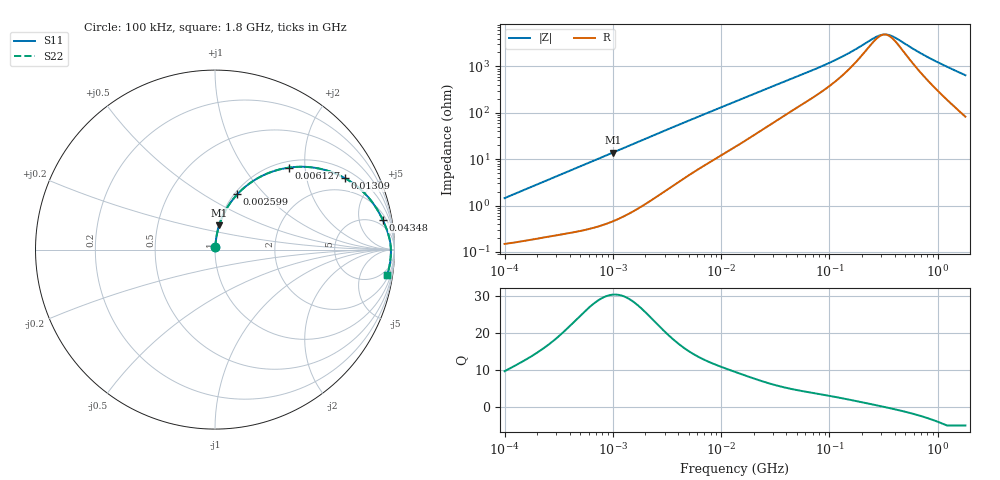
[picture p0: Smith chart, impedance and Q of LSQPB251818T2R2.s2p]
! LSQPB251818T2R2  S-PARAMETER MODEL  ( General Type )
! Model Generated by TAIYO YUDEN Corporation (http://www.ty-top.com)
! Version 2.0
! TAIYO YUDEN Control No. 100810NG19SB-FKC
! Copyright(c) 2009 TAIYO YUDEN CO.,LTD. All Rights Reserved.
! Product Description (link to TY-COMPAS)
! https://ds.yuden.co.jp/TYCOMPAS/or/detail?pn=LSQPB251818T2R2M&u=M
! Products Name : Inductors
! Characteristics :
!  Inductance : 2.2 uH , SRF(min) : 200 MHz , DC Resistance(max) : 0.156 Ohm
!  Rated Current : Saturation :1800 mA , Temp Rise : 1000 mA (40 degC)
!  Case Size : 2.5 x 1.8 / 0.098 x 0.071 [mm/inch] , Thickness : 1.8 / 0.071 [mm/inch]
!  (Conditions: Temperature = 25 degC , DC Bias Current/Voltage = 0A / 0V)
! External Node Assignments :
!  1  o---GGG---o  2
! GND o---------o GND
! Frequency Range : 0.1MHz  -  1800MHz  [ 402 STEP ]
# MHz S RI R 50
! Freq[MHz].  S11 Real  S11 Imag  S21 Real  S21 Imag  S12 Real  S12 Imag  S22 Real  S22 Imag
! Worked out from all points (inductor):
!   401 points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, 100 kHz to 1.8 GHz, reference 50 ohm
!   read as one part in series: L = 2.28 uH near 105 kHz
!   highest Q = 30.4 at 1 MHz (marker M1), where L = 2.21 uH
!   self-resonance near 322 MHz
!   S11 on the Smith chart (normalised r, x): 100 kHz: 1.00, +0.03; 2.599 MHz: 1.03, +0.71; 6.127 MHz: 1.12, +1.64; 13.09 MHz: 1.35, +3.38; 43.48 MHz: 3, +10; 1.8 GHz: 3, -13
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0.1  0.00169 0.0143  0.9983 -0.0143  0.9983 -0.0143  0.00169 0.0143
0.516129  0.00797 0.0712  0.992 -0.0712  0.992 -0.0712  0.00797 0.0712
0.999975  0.0232 0.1349  0.9768 -0.1349  0.9768 -0.1349  0.0232 0.1349
1.714072  0.0604 0.2207  0.9396 -0.2207  0.9396 -0.2207  0.0604 0.2207
2.59943  0.1241 0.308  0.8759 -0.308  0.8759 -0.308  0.1241 0.308
2.66389  0.1292 0.3134  0.8708 -0.3134  0.8708 -0.3134  0.1292 0.3134
3.942096  0.2367 0.3972  0.7633 -0.3972  0.7633 -0.3972  0.2367 0.3972
6.126528  0.41 0.4565  0.59 -0.4565  0.59 -0.4565  0.41 0.4565
8.84682  0.5715 0.4532  0.4285 -0.4532  0.4285 -0.4532  0.5715 0.4532
13.09176  0.7231 0.3985  0.2769 -0.3985  0.2769 -0.3985  0.7231 0.3985
13.41641  0.7312 0.3938  0.2688 -0.3938  0.2688 -0.3938  0.7312 0.3938
22.99727  0.8634 0.2803  0.1366 -0.2803  0.1366 -0.2803  0.8634 0.2803
43.47794  0.934 0.1668  0.066 -0.1668  0.066 -0.1668  0.934 0.1668
69.24595  0.9578 0.1092  0.0422 -0.1092  0.0422 -0.1092  0.9578 0.1092
137.4876  0.9743 0.0504  0.0257 -0.0504  0.0257 -0.0504  0.9743 0.0504
272.9811  0.9796 0.00896  0.0204 -0.00896  0.0204 -0.00896  0.9796 0.00896
316.1998  0.9799 0.00099  0.0201 -0.00099  0.0201 -0.00099  0.9799 0.00099
357.3983  0.9801 -0.00566  0.0199 0.00566  0.0199 0.00566  0.9801 -0.00566
413.9822  0.9801 -0.0138  0.0199 0.0138  0.0199 0.0138  0.9801 -0.0138
627.8136  0.979 -0.039  0.021 0.039  0.021 0.039  0.979 -0.039
863.2311  0.9766 -0.0626  0.0234 0.0626  0.0234 0.0626  0.9766 -0.0626
1800  0.9591 -0.1441  0.0409 0.1441  0.0409 0.1441  0.9591 -0.1441
